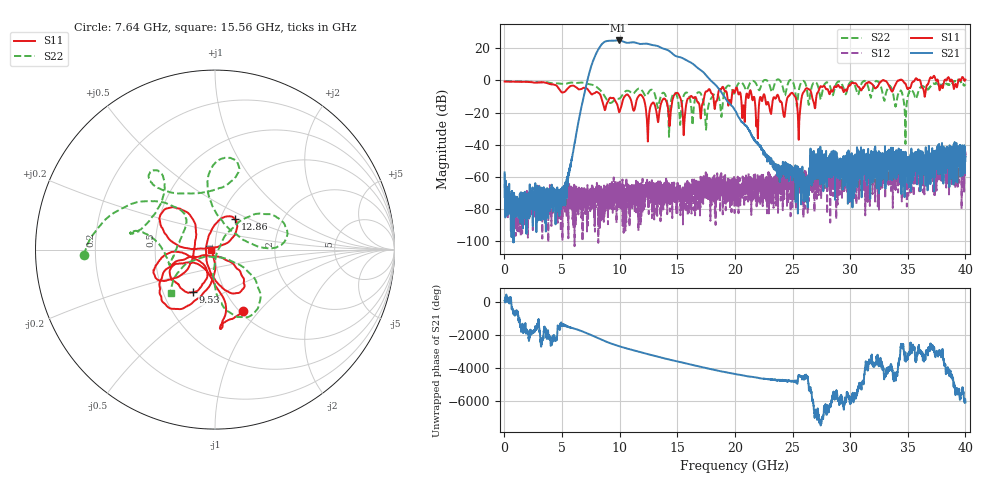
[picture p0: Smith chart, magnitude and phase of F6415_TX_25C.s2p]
!Keysight Technologies,N5245B,MY52451815,A.15.70.20
!Date: Thursday, April 18, 2024 09:59:52
!Correction: S33(C  2-Port  )
!S43(C  2-Port  )
!S34(C  2-Port  )
!S44(C  2-Port  )
!S2P File: Measurements: S33, S43, S34, S44:
# Hz S  RI  R 50
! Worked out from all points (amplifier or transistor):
!   4000 points, 10 MHz to 40 GHz, reference 50 ohm
!   highest |S21| = 24.9 dB at 9.9 GHz (marker M1)
!   |S21| within 3 dB of that: 8.371 GHz to 12.96 GHz (4.591 GHz wide, 43 % of centre)
!   unconditionally stable (mu >= 1): start of sweep to 22.5 GHz; 24.93 GHz to 32.78 GHz; 32.95 GHz to 34.14 GHz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
!   at 6.67 GHz: K = 11558.97, MAG = -9.4 dB, |S12| = -85.3 dB
!   at 20.01 GHz: K = 3621.30, MAG = -16.7 dB, |S12| = -62.5 dB
!   at 40 GHz: K = -1054.21, MSG = -1.7 dB, |S12| = -43.8 dB
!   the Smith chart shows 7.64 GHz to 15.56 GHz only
!   S11 on the Smith chart (normalised r, x): 7.64 GHz: 1.03, -0.82; 9.53 GHz: 0.71, -0.36; 12.86 GHz: 1.17, +0.41; 15.56 GHz: 0.96, -0.00
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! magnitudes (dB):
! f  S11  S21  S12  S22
! 10 MHz  -0.6  -57.2  -57.7  -0.5
! 720 MHz  -0.8  -80.8  -76.4  -0.6
! 4.92 GHz  -7.1  -80.1  -85.9  -2.0
! 6.68 GHz  -5.3  -16.4  -76.7  -1.3
! 7.64 GHz  -8.5  11.2  -77.2  -2.7
! 9.53 GHz  -11.5  24.8  -68.5  -12.2
! 9.9 GHz  -18.5  24.9  -76.1  -11.4
! 12.86 GHz  -13.9  22.0  -70.8  -6.1
! 13.34 GHz  -25.8  21.2  -73.7  -16.6
! 14.94 GHz  -7.7  15.0  -67.0  -9.1
! 15.56 GHz  -33.7  13.5  -73.4  -9.3
! 16.95 GHz  -17.3  6.8  -63.0  -7.5
! 17.52 GHz  -6.8  3.0  -73.0  -27.9
! 20.01 GHz  -6.9  -18.6  -62.5  -7.0
! 21.92 GHz  -25.0  -38.6  -68.6  -3.3
! 23.77 GHz  -9.8  -52.4  -62.8  0.6
! 25.55 GHz  -33.3  -55.2  -57.9  -5.9
! 26.2 GHz  -4.8  -63.9  -65.0  -3.9
! 26.67 GHz  -9.2  -57.1  -63.3  -3.8
! 33.34 GHz  -3.0  -46.4  -54.5  -3.6
! 34.79 GHz  -2.1  -51.5  -49.0  -37.5
! 40 GHz  0.6  -47.3  -43.8  -2.4
